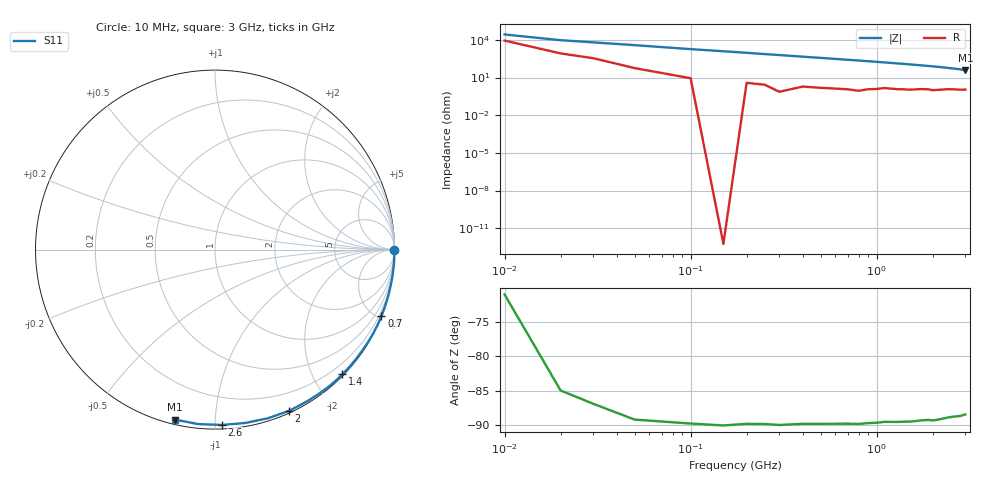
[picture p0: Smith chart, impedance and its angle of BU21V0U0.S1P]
! SIEMENS Small Signal Semiconductors
! BB833
! Si Tuning Diode in SOD323
! VR = 21 V
! S-Parameters:  April  1996
# GHz  S  MA  R  50
!  f  S11
! GHz  MAG  ANG
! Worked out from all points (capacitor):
!   31 points, 10 MHz to 3 GHz, reference 50 ohm
!   read as one part to ground: C = 836 fF near 10 MHz
!   lowest |Z| = 39.5 ohm at 3 GHz (marker M1)
!   S11 on the Smith chart (normalised r, x): 10 MHz: open; 700 MHz: 0.02, -5.22; 1.4 GHz: 0.02, -2.45; 2 GHz: 0.02, -1.56; 2.6 GHz: 0.02, -1.04; 3 GHz: 0.02, -0.79
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0.01  0.9988 -0.2
0.02  0.9991 -0.6
0.1  0.9997 -3.1
0.2  0.9996 -6.1
0.25  0.9995 -7.7
0.3  0.9998 -9.2
0.4  0.9991 -12.3
0.5  0.9989 -15.4
0.6  0.9986 -18.5
0.7  0.9983 -21.7
0.8  0.9984 -24.8
0.9  0.9972 -28.0
1  0.9964 -31.2
1.1  0.9949 -34.4
1.2  0.9945 -37.7
1.3  0.9942 -41.1
1.4  0.9933 -44.4
1.5  0.9929 -47.7
1.6  0.9916 -51.1
1.7  0.9899 -54.6
1.8  0.9887 -58.2
1.9  0.9879 -61.7
2  0.9886 -65.3
2.2  0.985 -72.6
2.4  0.9806 -80.0
2.6  0.9778 -87.8
2.8  0.9765 -95.5
3  0.9733 -103.4
